FUNCTION_BLOCK p07_ST_motor
VAR_INPUT
	naprej: BOOL;
	nazaj: BOOL;
	casBlokade: TIME;
END_VAR
VAR_OUTPUT
	premik: BOOL;
	smer: BOOL;
END_VAR
VAR
	casovnikNaprej: TOF;
	casovnikNazaj: TOF;
	vrtiNaprej: BOOL;
	vrtiNazaj: BOOL;
	blokadaNazaj: BOOL;
	blokadaNaprej: BOOL;
END_VAR


// Klic FB časovnikov
casovnikNaprej(IN:=naprej, PT:=casBlokade, Q => blokadaNazaj);
casovnikNazaj(IN:=nazaj, PT:=casBlokade, Q => blokadaNaprej);

// Izračun, ali lahko motor vrtimo naprej oziroma nazaj
vrtiNaprej := naprej AND NOT blokadaNaprej;
vrtiNazaj := nazaj AND NOT blokadaNazaj;

// Izhod premik
premik := vrtiNaprej OR vrtiNazaj;

// Izhod smer - želimo varčevati rele za smer,
// torej bomo pomnili stanje smeri.
(*
IF vrtiNazaj THEN
	smer := TRUE;
ELSIF vrtiNaprej THEN
	smer := FALSE;
ELSE               // To lahko 
	smer := smer;  // izpustimo.
END_IF
*)

// Krajše in slajše:
IF premik THEN
	smer := vrtiNazaj;
END_IF

END_FUNCTION_BLOCK
